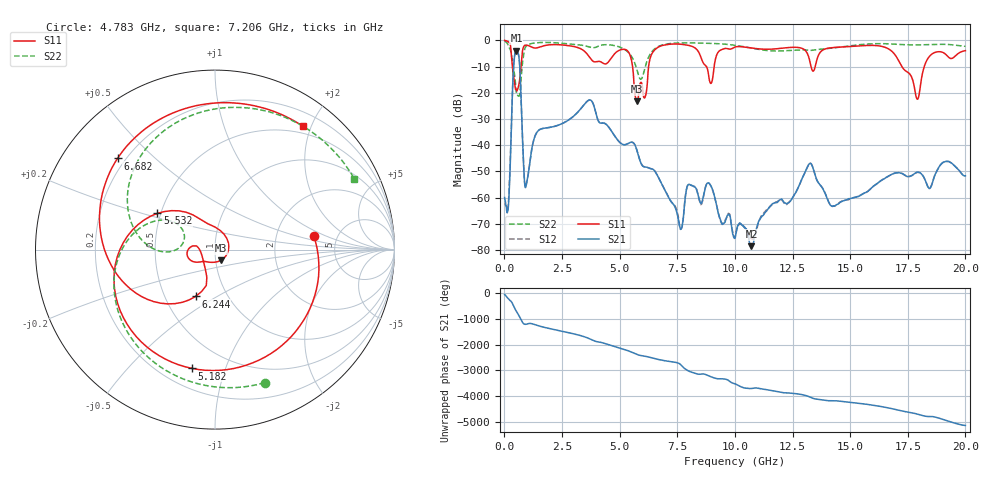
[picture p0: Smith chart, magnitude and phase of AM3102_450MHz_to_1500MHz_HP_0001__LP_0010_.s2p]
!Agilent Technologies,E8364B,MY43040894,A.07.50.67
!Agilent E8364B: A.07.50.67
!Date: Thursday, January 11, 2018 05:20:01
!Correction: S11(Full 2 Port(1,2))
!S21(Full 2 Port(1,2))
!S12(Full 2 Port(1,2))
!S22(Full 2 Port(1,2))
!S2P File: Measurements: S11, S21, S12, S22:
# Hz S  dB  R 50
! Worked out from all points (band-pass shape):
!   1601 points, 10 MHz to 20 GHz, reference 50 ohm
!   highest |S21| = -3.93 dB at 522.2 MHz (marker M1); lowest = -78.6 dB at 10.72 GHz (marker M2)
!   |S21| within 3 dB of the highest: 430.4 MHz to 638.9 MHz (208.5 MHz wide, 39 % of centre)
!   lowest |S11| = -23.3 dB at 5.757 GHz (marker M3), VSWR 1.15, Z = 52.9 - j6.41 ohm
!   |S11| at or under -10 dB: 347.9 MHz to 721 MHz (373.1 MHz wide, 69.8 % of centre); 5.56 GHz to 6.257 GHz (696.5 MHz wide, 11.8 % of centre); 17.24 GHz to 18.22 GHz (972.5 MHz wide, 5.48 % of centre)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
!   |S22| runs from -21.3 to -0.4 dB; largest |S21 - S12| = 0.0032
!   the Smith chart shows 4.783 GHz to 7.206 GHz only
!   S11 on the Smith chart (normalised r, x): 4.783 GHz: 3.32, +0.73; 5.182 GHz: 0.32, -0.77; 5.532 GHz: 0.48, +0.23; 6.244 GHz: 0.71, -0.40; 6.682 GHz: 0.17, +0.39; 7.206 GHz: 0.39, +1.87
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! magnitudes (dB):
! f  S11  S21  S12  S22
! 10 MHz  -0.1  -60.0  -62.3  -0.4
! 172.4 MHz  -0.6  -63.6  -62.3  -2.1
! 522.2 MHz  -18.9  -3.9  -3.9  -20.1
! 947 MHz  -1.8  -55.2  -55.2  -2.2
! 1.434 GHz  -2.8  -34.8  -34.8  -0.9
! 3.346 GHz  -3.4  -25.8  -25.8  -1.8
! 4.783 GHz  -5.1  -36.5  -36.5  -2.0
! 5.182 GHz  -3.4  -39.9  -39.9  -3.3
! 5.532 GHz  -8.4  -38.9  -38.9  -6.4
! 5.757 GHz  -23.3  -42.2  -42.2  -11.4
! 6.244 GHz  -11.0  -48.7  -48.6  -6.7
! 6.682 GHz  -2.6  -52.3  -52.3  -2.3
! 7.206 GHz  -1.5  -61.2  -61.2  -1.2
! 7.656 GHz  -1.5  -72.1  -72.1  -1.0
! 8.881 GHz  -14.6  -54.5  -54.6  -1.1
! 10.01 GHz  -2.5  -75.6  -75.2  -1.9
! 10.72 GHz  -2.9  -78.6  -75.7  -3.0
! 13.34 GHz  -11.1  -47.6  -47.6  -3.8
! 14.24 GHz  -2.8  -63.4  -63.3  -2.9
! 16.68 GHz  -3.3  -51.7  -51.7  -1.3
! 17.91 GHz  -22.5  -50.3  -50.4  -1.8
! 20 GHz  -4.0  -51.7  -51.8  -2.3
